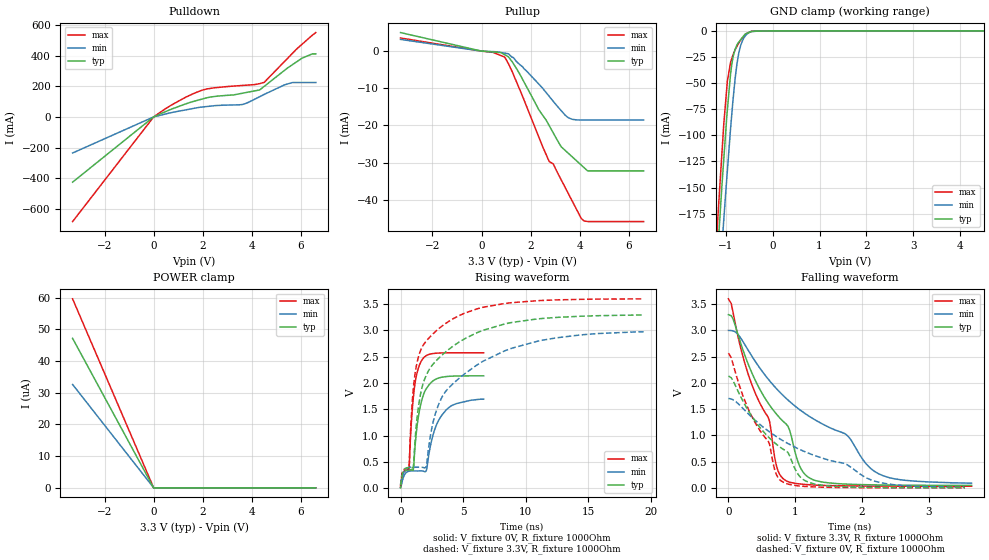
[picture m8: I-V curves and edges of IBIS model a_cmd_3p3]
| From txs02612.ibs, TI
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|   a_cmd_3p3 Model
[Model]   a_cmd_3p3
Model_type   I/O
Polarity   Non-Inverting
Enable   Active-High
Vinl = 0.15
Vinh = 3.1
Vmeas = 1.65
Vref = 1.65
Cref = 2pF
Rref = 1000
|   typ   min   max
|   (nom PVT)   (fast PVT)   (slow PVT)
|C_comp from frequency sweep method (F=30MHz)
C_comp   5.484e-12   5.367e-12   5.590e-12
|ON state : BUFFER OUTPUT TURNED HIGH
|C_comp   4.952e-12   4.724e-12   5.333e-12
|OFF state: BUFFER IN HIGH IMPEDANCE
|C_comp   5.484e-12   5.367e-12   5.590e-12
|C_comp from LC tank measurement(L=1nH)
|Average
|Resonant Frequency(Hz)   2.395e+09   2.435e+09   2.390e+09
|C_comp   4.421e-12   4.276e-12   4.439e-12
|ON state : BUFFER OUTPUT TURNED HIGH
|Resonant Frequency(Hz)   2.400e+09   2.440e+09   2.400e+09
|C_comp   4.402e-12   4.259e-12   4.402e-12
|OFF state: BUFFER IN HIGH IMPEDANCE
|Resonant Frequency(Hz)   2.390e+09   2.430e+09   2.380e+09
|C_comp   4.439e-12   4.294e-12   4.476e-12
[Model spec]
|subparameter
Vinl   0.15   0.15   0.15
Vinh   3.1   2.8   3.4
| Where nom  PVT is Nominal Process, 3.3V, 27C
|   Fast PVT is Strong Process,  3.6V, -40C
|   Slow PVT is Weak Process,   3V, 125C
[Voltage Range]   3.3   3   3.6
|Ambient Temperature   25   85   -40
|Junction Temperature
[Temperature Range]   27   125   -40
[Pullup Reference]   3.3   3   3.6
[Pulldown Reference]   0   0   0
[Power Clamp Reference]   3.3   3   3.6
[GND Clamp Reference]   0   0   0
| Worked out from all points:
|   slope of the pulldown table from 0 to 0.495 V, typ, clamps not added: 14.1 ohm
|   slope of the pullup table from 0 to 0.495 V, typ, clamps not added: 2.05 kohm
|   GND clamp passes 1 mA (typ) near -0.48 V on its own axis
|   falling waveform, V_fixture 3.3V, R_fixture 1000Ohm: 20-80 % time 783ps typ, 1.55ns min, 530ps max; typ from 3.3 V to 0.049 V
|   rising waveform, V_fixture 0V, R_fixture 1000Ohm: 20-80 % time 682ps typ, 1.14ns min, 488ps max; typ from 0.01 V to 2.14 V
|   rising waveform, V_fixture 3.3V, R_fixture 1000Ohm: 20-80 % time 2.78ns typ, 4.26ns min, 1.66ns max; typ from 0.054 V to 3.29 V
|   falling waveform, V_fixture 0V, R_fixture 1000Ohm: 20-80 % time 779ps typ, 1.55ns min, 524ps max; typ from 2.13 V to 0.004 V
[Pulldown]
|   Voltage   I(typ)   I(min)   I(max)
-3.3V     -425.6mA   -235.6mA   -682.8mA
0V        0A         0A         0A
1.246V    81.43mA    43.98mA    123.3mA
2.012V    118.1mA    65.01mA    176mA
3.621V    154.6mA    81.19mA    205.1mA
4.316V    175.9mA    131.7mA    217mA
4.504V    199.5mA    147mA      225.7mA
5.331V    304mA      209.1mA    362mA
5.649V    340.5mA    224.1mA    414.4mA
6.042V    383mA      224.1mA    473.9mA
6.455V    410.9mA    224.1mA    532.1mA
6.6V      411mA      224.1mA    550.1mA
[GND Clamp]
|   Voltage   I(typ)   I(min)   I(max)
-3.3V     -1.853A    -1.782A    -1.962A
-1.241V   -262mA     -314.6mA   -236.8mA
-1.163V   -206.8mA   -261.2mA   -175.8mA
-1.14V    -190.6mA   -245.6mA   -159.7mA
-1.044V   -125.3mA   -183.1mA   -91.85mA
-964.8mV  -76.15mA   -134.6mA   -48.64mA
-897.6mV  -42.03mA   -94.66mA   -30.57mA
-834.9mV  -23.5mA    -62.33mA   -22.02mA
-759mV    -13.51mA   -31.48mA   -14.82mA
-624mV    -5.265mA   -7.758mA   -5.889mA
-448.8mV  -403.5uA   -859.2uA   -460.2uA
6.6V      0A         0A         0A
[Pullup]
|   Voltage   I(typ)   I(min)   I(max)
-3.3V     4.985mA    3.143mA    3.53mA
478.8mV   -233.4uA   -139.6uA   -355.7uA
939.6mV   -956.7uA   -545.6uA   -1.596mA
1.399V    -4.44mA    -2.643mA   -7.914mA
2.32V     -15.65mA   -8.79mA    -22.95mA
2.747V    -19.95mA   -12.11mA   -29.6mA
2.916V    -21.96mA   -13.48mA   -30.33mA
3.241V    -25.71mA   -16mA      -34.59mA
3.549V    -27.57mA   -17.97mA   -38.52mA
4.057V    -30.64mA   -18.52mA   -44.99mA
4.316V    -32.2mA    -18.52mA   -45.83mA
6.6V      -32.2mA    -18.52mA   -45.83mA
[POWER Clamp]
|   Voltage   I(typ)   I(min)   I(max)
-3.3V     47.15uA    32.6uA     59.61uA
-66mV     945.1nA    676.6nA    1.197uA
-33.83fV  0A         10.17nA    0A
6.6V      0A         0A         0A
[Ramp]
R_load = 1000
|   typ   min   max
dV/dt_r   1.275/6.81249e-10   1.02013/1.1667e-09   1.53427/4.87487e-10
dV/dt_f   1.95137/7.83368e-10  1.75546/1.55434e-09   2.13807/5.30056e-10
[Falling Waveform]
V_fixture = 3.3V
V_fixture_min = 3V
V_fixture_max = 3.6V
R_fixture = 1000Ohm
|   Time   V(typ)   V(min)   V(max)
0s        3.299V     3V         3.6V
442ps     1.947V     2.334V     1.691V
617ps     1.576V     2.04V      1.265V
717ps     1.41V      1.894V     431.3mV
842ps     1.243V     1.733V     154.8mV
1.092ns   353.4mV    1.468V     74.46mV
1.292ns   146.4mV    1.301V     56.15mV
1.767ns   74.3mV     1.013V     40.58mV
2.317ns   57.4mV     234.1mV    35.97mV
3.642ns   48.56mV    92.02mV    33.86mV
[Rising Waveform]
V_fixture = 0V
V_fixture_min = 0V
V_fixture_max = 0V
R_fixture = 1000Ohm
|   Time   V(typ)   V(min)   V(max)
0s        10.22mV    5.581mV    15.52mV
192ps     266.2mV    179.9mV    293.5mV
667ps     346.7mV    322mV      332mV
1.017ns   348.7mV    328.2mV    1.707V
1.317ns   1.171V     326.7mV    2.187V
1.717ns   1.691V     327.2mV    2.44V
2.067ns   1.895V     341.2mV    2.521V
2.692ns   2.056V     1.089V     2.562V
3.617ns   2.121V     1.479V     2.573V
6.642ns   2.136V     1.691V     2.573V
[Rising Waveform]
V_fixture = 3.3V
V_fixture_min = 3V
V_fixture_max = 3.6V
R_fixture = 1000Ohm
|   Time   V(typ)   V(min)   V(max)
0s        54.08mV    76.41mV    46.3mV
192ps     311.9mV    252.9mV    326.1mV
667ps     391.8mV    394.4mV    367.9mV
1.017ns   400.2mV    399.1mV    1.872V
1.417ns   1.523V     397.3mV    2.483V
2.042ns   2.138V     410.7mV    2.793V
2.567ns   2.349V     1.22V      2.928V
3.292ns   2.525V     1.721V     3.078V
8.917ns   3.152V     2.663V     3.528V
19.42ns   3.292V     2.972V     3.599V
[Falling Waveform]
V_fixture = 0V
V_fixture_min = 0V
V_fixture_max = 0V
R_fixture = 1000Ohm
|   Time   V(typ)   V(min)   V(max)
0s        2.133V     1.705V     2.567V
242ps     1.595V     1.483V     1.673V
417ps     1.243V     1.27V      1.206V
592ps     979.9mV    1.09V      903.5mV
717ps     834.2mV    979.1mV    260mV
817ps     740.6mV    900.2mV    112.7mV
1.067ns   222.1mV    734.6mV    38.46mV
1.317ns   69.73mV    607.1mV    19.31mV
2.267ns   10.64mV    105.8mV    4.994mV
3.542ns   4.392mV    13.34mV    3.115mV
